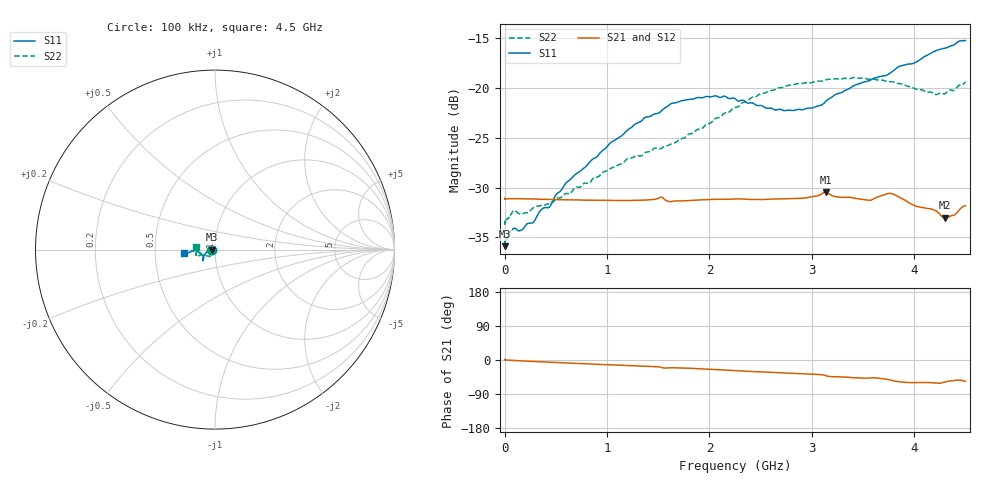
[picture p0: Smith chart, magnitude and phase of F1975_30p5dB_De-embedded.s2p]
! Integrated Device Technology
! Corporate Headquarters
! 6024 Silver Creek Valley Road
! San Jose, CA 95138  USA
! Phone:  1-408-284-8200
! Toll Free:  1-800-223-1366
! Webpage:  http://www.idt.com/
! Timing and RF Division
! 515 Groton Road, Suite 102
! Westford, MA 01886-6024
! Device:  F1975
! Description: 6-bit, 75 ohm, 0.5 dB Digital Step Attenuator
! Frequency:  5.0 MHz -  3.00 GHz
! Package:  4x4 mm QFN Plastic Package: 20 pin
! Ports:  2 RF, 11 DC
!  Pin  1  = D5 (16 dB)
!  Pin  2  = RF1  =  Port 1
!  Pin  3  = Serial Data In (DATA)
!  Pin  4  = Serial Clock (CLK)
!  Pin  5  = Serial Latch Enable (LE)
!  Pin  6  = VDD
!  Pin  7  = NC
!  Pin  8  = NC
!  Pin  9  = NC
!  Pin 10  = GND
!  Pin 11  = GND
!  Pin 12  = NC
!  Pin 13  = VMODE
!  Pin 14  = RF2  =  Port 2
!  Pin 15  = D4 (8 dB)
!  Pin 16  = D3 (4 dB)
!  Pin 17  = D2 (2 dB)
!  Pin 18  = NC
!  Pin 19  = D1 (1 dB)
!  Pin 20  = D0 (0.5 dB)
! State:  61
! Atten State:  30.5 dB
! Voltage:  +3.30 Volts
! Current:  0.560 mA
! Data:  The device was measured on a F1975 evaluation board which has
!  individual transmission lines to the RF pins.  Data was collected
!  using a calibrated network analyzer.  The evaluation board was
!  de-embedded using Automatic Fixture Removal (AFR).
!  The reference plane is the edge of the package pin.
! Misc:
!  Action Tracker AT0415
! Date Measured:  2018-02-08
! Date:  2018-03-26  MJV
! Note:
!  Integrated Device Technology supplies this data as a sample of measured
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# GHz S dB R 75
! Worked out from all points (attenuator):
!   291 points, 100 kHz to 4.5 GHz, reference 75 ohm
!   highest |S21| = -30.46 dB at 3.14 GHz (marker M1); lowest = -33.0 dB at 4.3 GHz (marker M2)
!   lowest |S11| = -35.9 dB at 100 kHz (marker M3), VSWR 1.03, Z = 72.6 - j0.00853 ohm
!   |S11| at or under -10 dB: start of sweep to end of sweep
!   |S22| runs from -33.8 to -19.0 dB; largest |S21 - S12| = 0.00013
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0.0001  -35.87 -179.8  -31.08 1.2  -31.07 1.2  -33.76 -179.1
0.006  -35.32 -178.4  -31.13 0.3  -31.15 0.5  -33.35 -177.8
0.08  -34.15 -176.2  -31.11 -1.0  -31.11 -1.0  -32.38 -169.6
0.16  -34.28 -177.2  -31.12 -2.2  -31.12 -2.2  -32.67 -160.1
0.28  -33.53 179.6  -31.15 -3.8  -31.15 -3.8  -32.02 -152.1
0.36  -32.20 179.8  -31.17 -4.8  -31.17 -4.8  -31.78 -144.6
0.44  -31.95 -179.5  -31.19 -5.8  -31.18 -5.8  -31.71 -139.0
0.5  -30.73 -179.7  -31.20 -6.5  -31.20 -6.6  -31.17 -138.3
0.6  -29.53 -176.0  -31.22 -7.8  -31.22 -7.8  -30.59 -133.1
0.76  -28.18 -169.4  -31.25 -9.7  -31.25 -9.6  -29.71 -129.1
1.28  -23.60 -153.1  -31.28 -15.4  -31.27 -15.4  -26.80 -124.8
1.52  -22.43 -145.1  -30.98 -18.6  -30.97 -18.6  -26.13 -131.3
1.62  -21.62 -143.4  -31.41 -20.6  -31.41 -20.5  -25.67 -134.7
1.88  -20.99 -139.5  -31.26 -22.7  -31.26 -22.7  -24.19 -147.2
2.26  -21.17 -138.5  -31.15 -28.1  -31.15 -28.1  -21.95 -158.0
2.64  -22.22 -147.9  -31.15 -33.0  -31.14 -33.0  -20.19 -159.5
3.02  -21.97 -164.3  -30.88 -37.6  -30.87 -37.6  -19.42 -160.2
3.14  -21.31 -167.0  -30.46 -41.7  -30.46 -41.7  -19.19 -160.7
3.56  -19.30 -177.5  -31.28 -47.7  -31.28 -47.7  -19.15 -166.2
3.76  -18.57 -176.2  -30.58 -52.5  -30.58 -52.5  -19.39 -169.9
4.3  -16.04 -173.1  -33.03 -58.4  -33.03 -58.3  -20.61 177.0
4.5  -15.26 -172.8  -31.81 -56.2  -31.81 -56.3  -19.41 173.4
